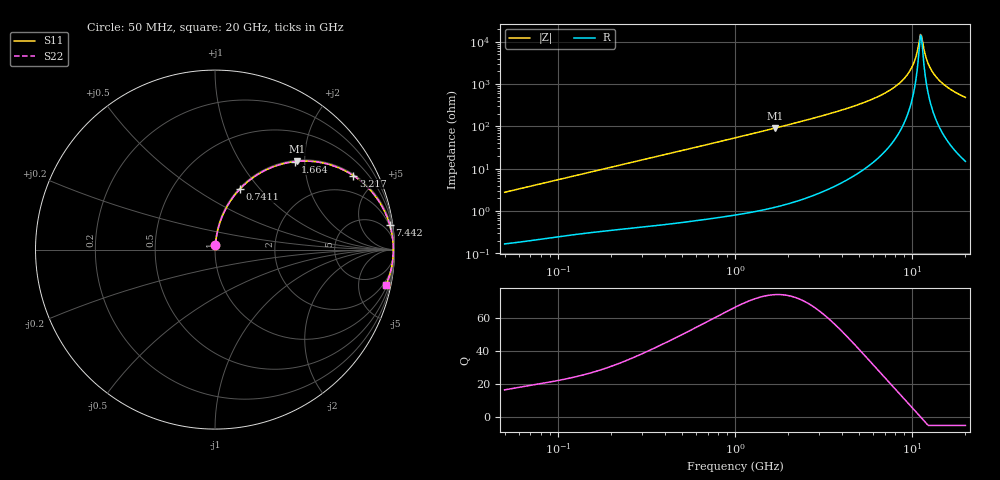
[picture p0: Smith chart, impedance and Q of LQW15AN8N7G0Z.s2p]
!Murata Part Number: LQW15AN8N7G0Z
!These Parameters are Measured in Series Mode Connection
!  o--[Z]--o
!Port1  Port2
!  o-------o
!Freq. Start=50[MHz] Stop=20[GHz], 401[Steps]
# Hz S RI R 50
!Freq.(Hz) S11(Real) S11(Imag) S21(Real) S21(Imag) S12(Real) S12(Imag) S22(Real) S22(Imag)
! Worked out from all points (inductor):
!   401 points, 50 MHz to 20 GHz, reference 50 ohm
!   read as one part in series: L = 8.76 nH near 51.52 MHz
!   highest Q = 74.2 at 1.689 GHz (marker M1), where L = 8.61 nH
!   self-resonance near 11.15 GHz
!   S11 on the Smith chart (normalised r, x): 50 MHz: 1.00, +0.06; 741.1 MHz: 1.01, +0.79; 1.664 GHz: 1.02, +1.80; 3.217 GHz: 1.06, +3.70; 7.442 GHz: 2, +14; 20 GHz: 1.30, -9.66
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5e7  0.00243 0.0275  0.9976 -0.0275  0.9976 -0.0275  0.00243 0.0275
1.364002e8  0.00829 0.0731  0.9917 -0.0731  0.9917 -0.0731  0.00829 0.0731
3.721004e8  0.0421 0.1896  0.9579 -0.1896  0.9579 -0.1896  0.0421 0.1896
7.411344e8  0.1392 0.3378  0.8608 -0.3378  0.8608 -0.3378  0.1392 0.3378
1e9  0.2254 0.4104  0.7746 -0.4104  0.7746 -0.4104  0.2254 0.4104
1.664083e9  0.448 0.4906  0.552 -0.4906  0.552 -0.4906  0.448 0.4906
1.689197e9  0.4557 0.4913  0.5443 -0.4913  0.5443 -0.4913  0.4557 0.4913
2.728004e9  0.6985 0.4516  0.3015 -0.4516  0.3015 -0.4516  0.6985 0.4516
3.216634e9  0.7705 0.4125  0.2295 -0.4125  0.2295 -0.4125  0.7705 0.4125
5.273168e9  0.9218 0.2559  0.0782 -0.2559  0.0782 -0.2559  0.9218 0.2559
7.442007e9  0.9738 0.1376  0.0262 -0.1376  0.0262 -0.1376  0.9738 0.1376
8.644534e9  0.9857 0.0869  0.0143 -0.0869  0.0143 -0.0869  0.9857 0.0869
9.600142e9  0.9907 0.0517  0.00926 -0.0517  0.00926 -0.0517  0.9907 0.0517
1.034674e10  0.9928 0.0267  0.00724 -0.0267  0.00724 -0.0267  0.9928 0.0267
1.098561e10  0.9935 0.00667  0.00654 -0.00667  0.00654 -0.00667  0.9935 0.00667
1.115139e10  0.9935 0.00167  0.0065 -0.00167  0.0065 -0.00167  0.9935 0.00167
1.149051e10  0.9934 -0.00832  0.00655 0.00832  0.00655 0.00832  0.9934 -0.00832
1.201863e10  0.993 -0.0233  0.00701 0.0233  0.00701 0.0233  0.993 -0.0233
1.238412e10  0.9924 -0.0333  0.00757 0.0333  0.00757 0.0333  0.9924 -0.0333
1.354865e10  0.9895 -0.0634  0.0105 0.0634  0.0105 0.0634  0.9895 -0.0634
1.597544e10  0.9791 -0.119  0.0209 0.119  0.0209 0.119  0.9791 -0.119
2e10  0.9534 -0.196  0.0466 0.196  0.0466 0.196  0.9534 -0.196
